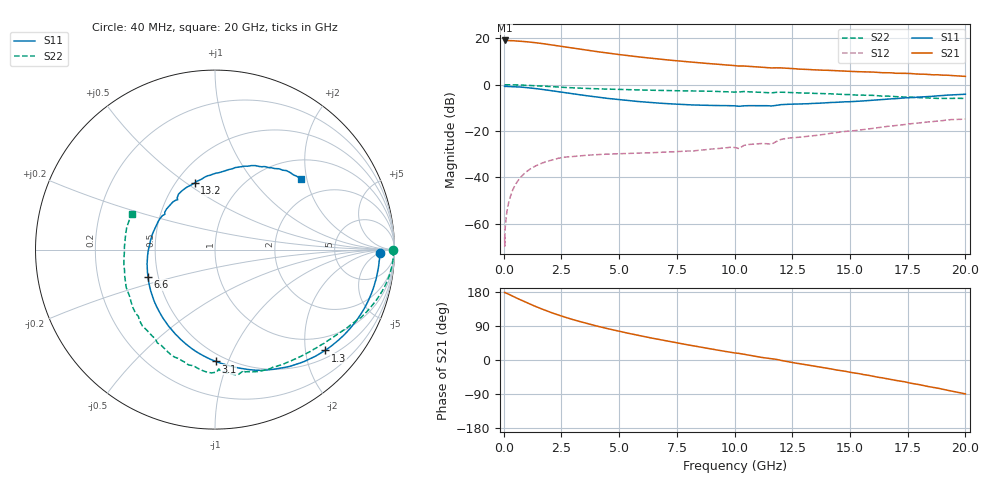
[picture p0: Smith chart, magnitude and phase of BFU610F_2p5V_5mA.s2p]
! Filename:  P:\Prog\Test\Noise\ATS_data\Testdata_Net\SplitFiles\BFU610_2W_A5_HighFreq_2.5V_5mA_D.s2p
! Date/Time: Wed 10/Aug/2011 16:55:25
! BFU610_2W_A5_HighFreq_Bias4_2.5V_1mA_10mA_R.s2p
! MDIF S-parameter v. bias file
! BFU610_2W_A5_HighFreq_2.5V_1mA_10mA
! Date/time Mon Aug 08 14:04:20 2011
! VAR V_out= 2.5000
! VAR I_out= 4.9900
! VAR V_in= 0.8966
! VAR I_in= 0.0402
! Device data file deembeded for feedlines and parallel
! Original file: \SplitFiles\BFU610_2W_A5_HighFreq_2.5V_5mA_R.s2p
! Feed-files: PR003V01_101208_Feed1.s2p, PR003V01_101208_Feed2.s2p
! Parallel-file: PR003V01_101208_Par.s2p
# MHz S MA R 50
!  Freq-MHz  S11-mag  S11-arg  S21-mag  S21-arg  S12-mag  S12-arg  S22-mag  S22-arg
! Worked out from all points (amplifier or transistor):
!   167 points, 40 MHz to 20 GHz, reference 50 ohm
!   highest |S21| = 19.1 dB at 40 MHz (marker M1)
!   |S21| within 3 dB of that: start of sweep to 2.788 GHz
!   unconditionally stable (mu >= 1): 4.923 GHz to 17.3 GHz
!   at 550 MHz: K = 0.05, MSG = 30.7 dB, |S12| = -42.4 dB
!   at 4.2 GHz: K = 0.84, MSG = 22.1 dB, |S12| = -30.1 dB
!   at 20 GHz: K = 0.82, MSG = 9.2 dB, |S12| = -14.8 dB
!   S11 on the Smith chart (normalised r, x): 40 MHz: 22, -6; 1.3 GHz: 0.66, -2.42; 3.1 GHz: 0.44, -0.90; 6.6 GHz: 0.44, -0.16; 13.2 GHz: 0.62, +0.54; 20 GHz: 1.45, +1.85
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40  0.9173 -1.3  8.967 178.4  0.0005134 87.0  0.992 -0.3
50  0.9097 -1.9  8.931 178.4  0.000329 119.9  0.9922 -0.4
60  0.918 -1.7  8.95 177.6  0.0007641 104.7  0.9934 -0.5
160  0.9166 -5.4  8.893 175.2  0.002114 88.9  0.9938 -1.9
380  0.909 -12.9  8.848 168.7  0.005193 85.6  0.9909 -4.8
800  0.8814 -26.9  8.595 156.7  0.0109 76.2  0.9767 -10.0
1300  0.8316 -42.5  8.111 143.3  0.01683 66.3  0.9512 -15.6
1700  0.7853 -54.2  7.652 133.5  0.02065 59.5  0.9284 -19.7
2050  0.7427 -63.9  7.227 125.4  0.02328 54.3  0.909 -23.0
2500  0.6871 -75.6  6.671 116.0  0.02651 48.5  0.8794 -26.9
3100  0.6229 -89.6  5.996 104.8  0.02846 42.0  0.8502 -31.4
3400  0.5944 -96.4  5.707 99.8  0.02943 40.1  0.8367 -33.5
4100  0.5346 -111.2  5.103 88.7  0.03116 36.2  0.8117 -38.1
4900  0.4804 -126.8  4.518 77.2  0.03225 33.6  0.7895 -43.4
6600  0.403 -157.9  3.615 55.7  0.03438 32.7  0.7535 -54.4
6800  0.3971 -161.4  3.526 53.3  0.03465 33.0  0.751 -55.7
8600  0.3603 169.0  2.931 33.2  0.0389 37.4  0.7259 -67.6
10200  0.3414 144.8  2.517 17.4  0.04181 42.0  0.6951 -77.2
13200  0.3881 106.9  2.122 -13.6  0.07666 37.1  0.659 -103.0
13400  0.3941 104.8  2.091 -15.6  0.07907 36.3  0.6491 -105.2
16800  0.4939 70.4  1.798 -51.6  0.1284 17.4  0.56 -144.8
20000  0.621 39.3  1.505 -89.4  0.1816 -14.0  0.5047 157.0
